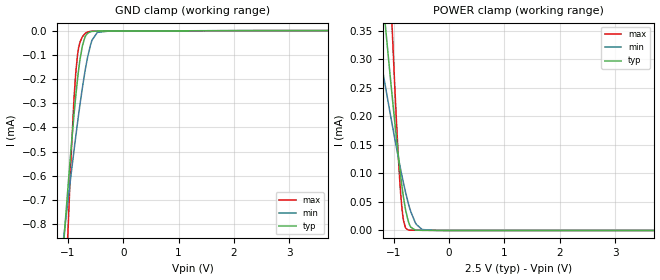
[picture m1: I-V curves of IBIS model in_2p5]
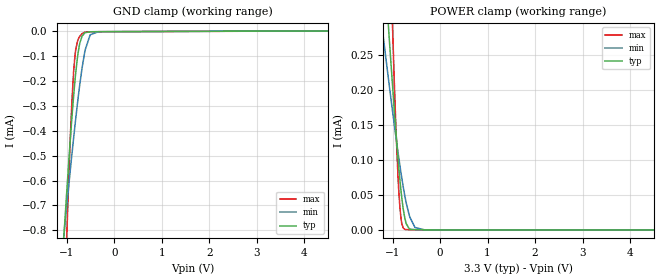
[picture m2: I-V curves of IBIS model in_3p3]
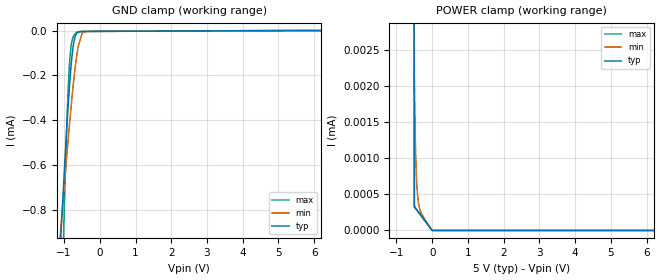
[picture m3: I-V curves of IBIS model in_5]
|Texas Instruments Incorporated
| High-Performance, 8000 VPK Reinforced Dual Channel Digital Isolator
| Marketing part#   Digital Voltage Range   Package-type   #pins
| ISO7820DW   2.25V-5.5V   SOIC   16
| ISO7820DWW   2.25V-5.5V   SOIC   16
[IBIS Ver]   4.1
[File name]   iso7820.ibs
[File Rev]   1.1
[Date]   5/12/2016
[Source]
| Texas Instruments Incorporated.
| Analog-eLab Design Center, HPA
| 12500 TI Blvd
| Dallas, TX -75243
[Notes]   Revision History:
| Rev 1.1: 5/12/2016
| - Add DWW package component
| Rev 1.0: 7/2/2015
| - Initial version of the model
| - Model generated from simulations in TISPICE
| - Model matched to SPICE simulation
| - C_comp although listed in numerical order of value are
|   obtained from varying PVT conditions. For PVT conditions for
|   each specific value refer the buffer description under
|   respective [Model]. IBIS model user is responsible for using
|   appropriate C_comp to simulate for Signal Integrity.
| - This is relative part of ISO7841.
|* EXCEPTION:   *
|* - For in_* models there will be leakage current in GROUND clamp  *
|*   because of a resistor(RH2) connected to pad.   *
[Disclaimer]
| This model is designed as an aid for customers of Texas Instruments.
| TI and its licensors and suppliers make no warranties, either expressed
| or implied, with respect to this  model, including the warranties of
| merchantability or fitness for a particular purpose. The model is
| provided solely on an "as is" basis. The entire risk as to its quality
| and performance is with the customer.
[Copyright]
(C) Copyright 2016 Texas Instruments Incorporated.All rights reserved.
|   IS07820DW
[Component]   IS07820DW
[Manufacturer]   TI
[Package]   |16 SOIC - DW package
|   typ   min   max
R_pkg   0.12558   0.1249   0.12620
L_pkg   1.93563nH   1.9245nH   1.94750nH
C_pkg   0.4209pF   0.3263pF   0.6128pF
[Pin]  signal_name   model_name   R_pin   L_pin   C_pin
1   GND1   GND   0.0970   2.2582nH   0.6389pF
2   NC   NC   0.1057   2.1519nH   0.3071pF
3   VCC1   POWER   0.1289   1.9955nH   0.2145pF
4   INA   IN   0.1250   1.9245nH   0.3778pF
5   INB   IN   0.1249   1.9265nH   0.3667pF
6   NC   NC   0.1404   2.1876nH   0.4324pF
7   GND1   GND   0.1781   2.8364nH   0.4590pF
8   NC   NC   0.0822   2.4395nH   0.4450pF
9   GND2   GND   0.1013   2.4407nH   0.4093pF
10   NC   NC   0.1793   2.8571nH   0.5272pF
11   NC   NC   0.1288   1.9962nH   0.5084pF
12   OUTB   OUT   0.1262   1.9440nH   0.3263pF
13   OUTA   OUT   0.1262   1.9475nH   0.6128pF
14   VCC2   POWER   0.1405   2.1861nH   0.3810pF
15   NC   NC   0.0827   2.0901nH   0.7509pF
16   GND2   GND   0.0975   2.2691nH   0.6744pF
|   IS07820DWW
[Component]   IS07820DWW
[Manufacturer]   TI
[Package]   |16 SOIC - DWW package
|   typ   min   max
R_pkg   0.2986   0.2007   0.3729
L_pkg   6.1920nH   5.7068nH   6.9814nH
C_pkg   0.3776pF   0.0527pF   0.7658pF
[Pin]  signal_name   model_name   R_pin   L_pin   C_pin
1   GND1   GND   0.2515   6.9814nH   0.7658pF
2   NC   NC   0.2414   6.4743nH   0.4827pF
3   VCC1   POWER   0.3404   6.2419nH   0.3712pF
4   INA   IN   0.2997   5.8575nH   0.3661pF
5   INB   IN   0.3048   5.7068nH   0.3697pF
6   NC   NC   0.3229   5.9972nH   0.3885pF
7   GND1   GND   0.3729   6.6301nH   0.3885pF
8   NC   NC   0.2162   5.8346nH   0.4827pF
9   GND2   GND   0.2007   6.5823nH   0.5517pF
10   NC   NC   0.3456   6.8632nH   0.3887pF
11   NC   NC   0.3109   6.1891nH   0.3704pF
12   OUTB   OUT   0.2997   5.7473nH   0.3669pF
13   OUTA   OUT   0.3032   5.8251nH   0.3710pF
14   VCC2   POWER   0.3351   6.1684nH   0.0527pF
15   NC   NC   0.2007   5.7509nH   0.5517pF
16   GND2   GND   0.2768   6.8945nH   0.0527pF
|   Model Selectors
[Model Selector] IN
in_2p5   2.5V digital Input
in_3p3   3.3V digital Input
in_5   5.0V digital Input
[Model Selector] OUT
out_2p5   2.5V digital 3-state
out_3p3   3.3V digital 3-state
out_5   5.0V digital 3-state
| Models and submodels in the file (6): in_2p5 (Input), in_3p3 (Input), in_5 (Input), out_2p5 (3-state), out_3p3 (3-state), out_5 (3-state)
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|   in_2p5 Model
[Model]   in_2p5
Model_type   Input
Vinl = 0.75
Vinh = 1.75
|   typ   min   max
|   (nom PVT)   (fast PVT)   (slow PVT)
C_comp   3.281e-15   3.281e-15   3.250e-14
[Model spec]
|subparameter
Vinl   0.75   0.675   0.825
Vinh   1.75   1.575   1.925
| Where nom  PVT is Nominal Process, 2.5V, 27C
|   Fast PVT is Strong Process,  2.75V, -55C
|   Slow PVT is Weak Process,   2.25V, 150C
[Voltage Range]   2.5   2.25   2.75
|Ambient Temperature   25   125   -55
|Junction Temperature
[Temperature Range]   27   150   -55
[Power Clamp Reference]   2.5   2.25   2.75
[GND Clamp Reference]   0   0   0
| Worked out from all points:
|   GND clamp passes 1 mA (typ) near -1.12 V on its own axis
[GND Clamp]
|   Voltage   I(typ)   I(min)   I(max)
-2.5V     -5.567mA   -3.855mA   -11.2mA
-1.071V   -859.9uA   -843.3uA   -1.249mA
-1.015V   -691.9uA   -732.5uA   -914.2uA
-965mV    -547.7uA   -635.6uA   -635.6uA
-894mV    -356.2uA   -501.7uA   -297uA
-827.5mV  -201.6uA   -381.9uA   -101.5uA
-737.5mV  -61.36uA   -233.7uA   -24.74uA
-643.8mV  -10.62uA   -108.8uA   -5.86uA
-564mV    -3.337uA   -39.15uA   -2.62uA
-468.2mV  -2.078uA   -7.417uA   -2.095uA
-250mV    -1.826uA   -1.892uA   -1.932uA
5V        0A         0A         0A
[POWER Clamp]
|   Voltage   I(typ)   I(min)   I(max)
-2.5V     1.812mA    1.039mA    3.985mA
-1.351V   565.2uA    364.2uA    1.113mA
-1.196V   404.1uA    277.3uA    740.6uA
-1.053V   258.8uA    198.6uA    407.1uA
-990.2mV  197.6uA    165uA      269.2uA
-924.3mV  136.7uA    131uA      139.5uA
-874.8mV  94.88uA    106.6uA    63.72uA
-822.5mV  56.84uA    82.23uA    17.11uA
-740mV    16.82uA    48.51uA    910.2nA
-612.5mV  771.4nA    14.03uA    395.2nA
-486.3mV  326.4nA    1.63uA     313.2nA
5V        0A         0A         0A
|   in_3p3 Model
[Model]   in_3p3
Model_type   Input
Vinl = 0.99
Vinh = 2.31
|   typ   min   max
|   (nom PVT)   (fast PVT)   (slow PVT)
C_comp   3.281e-15   3.281e-15   3.329e-14
[Model spec]
|subparameter
Vinl   0.99   0.891   1.089
Vinh   2.31   2.079   2.541
| Where nom  PVT is Nominal Process, 3.3V, 27C
|   Fast PVT is Strong Process,  3.63V, -55C
|   Slow PVT is Weak Process,   2.97V, 150C
[Voltage Range]   3.3   2.97   3.63
|Ambient Temperature   25   125   -55
|Junction Temperature
[Temperature Range]   27   150   -55
[Power Clamp Reference]   3.3   2.97   3.63
[GND Clamp Reference]   0   0   0
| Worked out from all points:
|   GND clamp passes 1 mA (typ) near -1.12 V on its own axis
|   POWER clamp passes 1 mA (typ) near -1.76 V on its own axis
[GND Clamp]
|   Voltage   I(typ)   I(min)   I(max)
-3.3V     -8.284mA   -5.57mA    -16.97mA
-1.076V   -873.8uA   -852.4uA   -1.277mA
-1.002V   -654.6uA   -707.6uA   -841.1uA
-893.3mV  -354.6uA   -500.5uA   -294.5uA
-853.4mV  -258.1uA   -427.8uA   -159.9uA
-825mV    -196.7uA   -377.6uA   -97.46uA
-772.2mV  -104.4uA   -288.5uA   -41.12uA
-722.7mV  -47.98uA   -211.7uA   -20.38uA
-620.4mV  -7.55uA    -84.56uA   -4.818uA
-505.2mV  -2.819uA   -14.66uA   -2.744uA
-330mV    -2.413uA   -2.673uA   -2.551uA
6.6V      0A         0A         0A
[POWER Clamp]
|   Voltage   I(typ)   I(min)   I(max)
-3.3V     2.693mA    1.517mA    6.009mA
-1.242V   451.1uA    302.7uA    849uA
-1.198V   405.5uA    278.1uA    743.9uA
-1.049V   255uA      196.5uA    398.4uA
-965.9mV  174.7uA    152.3uA    218.9uA
-878.8mV  98.13uA    108.5uA    68.84uA
-842.5mV  70.44uA    91.34uA    30.66uA
-805.2mV  46.22uA    74.6uA     9.403uA
-737.2mV  15.94uA    47.51uA    852.4nA
-526mV    364.9nA    3.505uA    338.9nA
-330mV    219.3nA    268.9nA    212.6nA
6.6V      0A         0A         0A
|   in_5 Model
[Model]   in_5
Model_type   Input
Vinl = 1.5
Vinh = 3.5
|   typ   min   max
|   (nom PVT)   (fast PVT)   (slow PVT)
C_comp   3.281e-15   3.281e-15   3.455e-14
[Model spec]
|subparameter
Vinl   1.5   1.35   1.65
Vinh   3.5   3.15   3.85
| Where nom  PVT is Nominal Process, 5V, 27C
|   Fast PVT is Strong Process,  5.5V, -55C
|   Slow PVT is Weak Process,   4.5V, 150C
[Voltage Range]   5   4.5   5.5
|Ambient Temperature   25   125   -55
|Junction Temperature
[Temperature Range]   27   150   -55
[Power Clamp Reference]   5   4.5   5.5
[GND Clamp Reference]   0   0   0
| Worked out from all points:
|   GND clamp passes 1 mA (typ) near -1.12 V on its own axis
[GND Clamp]
|   Voltage   I(typ)   I(min)   I(max)
-5V       -13.99mA   -9.044mA   -29.25mA
-1.112V   -984.6uA   -924.8uA   -1.503mA
-1.062V   -832.2uA   -825.1uA   -1.194mA
-974mV    -573.5uA   -653.1uA   -684.8uA
-908mV    -392.7uA   -527.9uA   -356.7uA
-850mV    -250.8uA   -421.9uA   -151.8uA
-809mV    -166.1uA   -350.2uA   -74.38uA
-740mV    -65.1uA    -237.9uA   -26.95uA
-608mV    -7.374uA   -73.42uA   -5.426uA
-500mV    -3.903uA   -14.37uA   -3.931uA
-338mV    -3.55uA    -3.864uA   -3.762uA
10V       0A         0A         0A
[POWER Clamp]
|   Voltage   I(typ)   I(min)   I(max)
-5V       185.5mA    66.86mA    305.6mA
-1.007V   213.6uA    173.9uA    305uA
-500mV    338.3nA    2.124uA    322.2nA
-482mV    323.5nA    1.505uA    310.6nA
-473mV    316.7nA    1.273uA    304.8nA
-459.5mV  306.8nA    1.002uA    296.1nA
-432.5mV  288nA      655.7nA    278.7nA
-396.5mV  263.7nA    427.3nA    255.5nA
-360.5mV  239.7nA    320.4nA    232.3nA
-306.5mV  203.8nA    241.2nA    197.5nA
-500uV    0A         0A         0A
10V       0A         0A         0A
